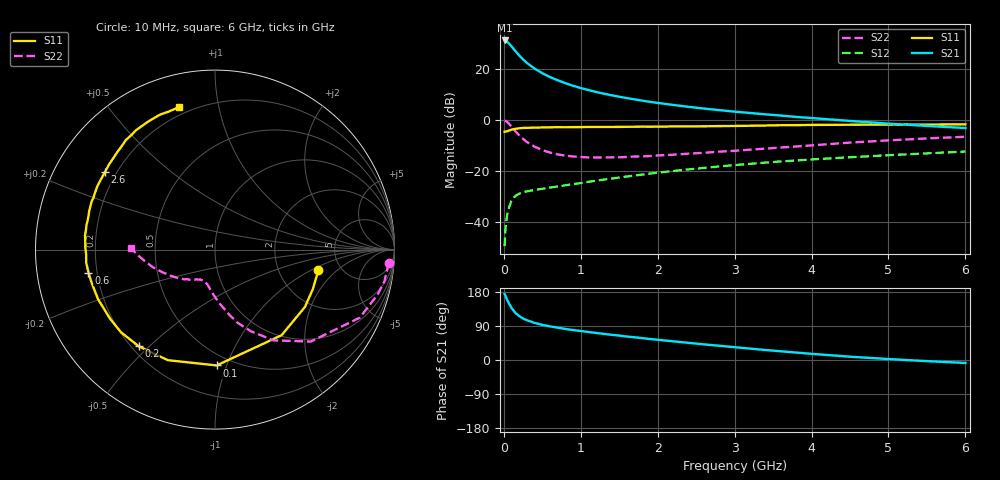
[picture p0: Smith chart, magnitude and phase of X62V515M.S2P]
! SIEMENS Small Signal Semiconductors
! BFP193W
! Si NPN RF Bipolar Junction Transistor in SOT343
! VCE = 2.5 V  IC = 15 mA
! Common Emitter S-Parameters:  April 1994
# GHz  S  MA  R  50
!  f  S11  S21  S12  S22
! GHz  MAG  ANG  MAG  ANG  MAG  ANG  MAG  ANG
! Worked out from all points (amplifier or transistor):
!   40 points, 10 MHz to 6 GHz, reference 50 ohm
!   highest |S21| = 31.1 dB at 10 MHz (marker M1)
!   |S21| within 3 dB of that: start of sweep to 119 MHz
!   unconditionally stable (mu >= 1): 1.109 GHz to 3.98 GHz
!   at 200 MHz: K = 0.29, MSG = 27.0 dB, |S12| = -28.8 dB
!   at 1.5 GHz: K = 1.11, MAG = 13.8 dB, |S12| = -22.5 dB
!   at 6 GHz: K = 0.93, MSG = 4.6 dB, |S12| = -12.4 dB
!   S11 on the Smith chart (normalised r, x): 10 MHz: 3.41, -1.18; 100 MHz: 0.42, -0.92; 200 MHz: 0.23, -0.46; 600 MHz: 0.17, -0.09; 2.6 GHz: 0.16, +0.31; 6 GHz: 0.16, +0.77
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0.01  0.5876 -11.1  35.76 174.0  0.0034 86.1  0.9713 -4.4
0.02  0.5879 -22.1  35.56 169.8  0.0071 79.1  0.9603 -10.6
0.03  0.5944 -32.5  35.03 165.0  0.0102 77.8  0.9399 -15.5
0.05  0.6043 -52.1  33.19 155.6  0.0162 69.3  0.8913 -25.2
0.1  0.6454 -89.2  27.43 137.3  0.0268 54.0  0.7394 -43.9
0.15  0.6698 -113.1  22.19 124.4  0.0327 45.3  0.6014 -57.2
0.2  0.6863 -128.3  18.15 115.8  0.0361 40.0  0.4987 -66.1
0.25  0.6975 -138.8  15.28 109.6  0.0385 37.3  0.4265 -72.9
0.3  0.7001 -146.7  13.02 104.9  0.0401 36.0  0.3689 -77.8
0.4  0.7077 -157.0  10.08 97.9  0.0427 35.4  0.2995 -85.4
0.5  0.7115 -164.5  8.198 92.7  0.0451 36.2  0.2573 -91.0
0.6  0.7165 -169.7  6.879 88.6  0.0477 37.4  0.2299 -95.6
0.8  0.7181 -177.7  5.22 82.0  0.0527 40.6  0.2004 -101.9
1.1  0.7286 173.9  3.841 73.9  0.0617 44.9  0.1846 -109.4
1.3  0.7288 169.0  3.254 68.9  0.0681 47.1  0.1845 -113.0
1.6  0.7337 162.5  2.671 61.9  0.0782 49.1  0.1884 -117.7
2.2  0.7449 151.7  1.964 49.3  0.1002 50.5  0.2088 -127.2
2.6  0.7498 144.8  1.668 41.2  0.1152 50.0  0.2273 -133.5
3.2  0.769 135.1  1.366 30.1  0.1384 48.0  0.262 -143.1
4.5  0.8046 117.6  0.955 8.7  0.1862 41.1  0.36 -164.2
5.5  0.8109 108.7  0.762 -3.0  0.2217 35.4  0.4344 -176.3
6  0.8186 104.2  0.695 -7.8  0.2406 32.6  0.4687 178.9
